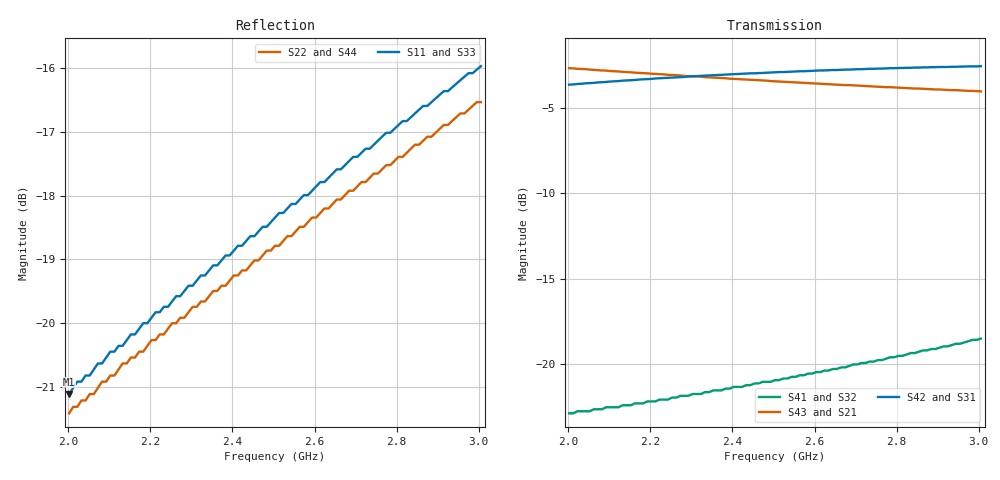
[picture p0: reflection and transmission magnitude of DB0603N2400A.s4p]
!	AVX THIN FILM OPERATION
!	0603 SIZE 3dB 90deg COUPLER P/N DB0603N2400ANTR
!	Created August 2007
!	Network Analyzer HP8720E S.07.64: Feb23, 2000 Serial No.US39172382
#	MHZ	S	MA	R	50
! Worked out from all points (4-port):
!   101 points, 2.003 GHz to 3.005 GHz, reference 50 ohm
!   strongest paths, dB at 2.003 GHz, 2.253 GHz, 2.504 GHz, 2.754 GHz, 3.005 GHz:
!     S42: -3.6, -3.2, -2.9, -2.7, -2.6
!     S31: -3.8, -3.4, -3.1, -3.0, -2.9
!     S43: -2.7, -3.1, -3.5, -3.8, -4.0
!     S21: -2.7, -3.1, -3.5, -3.8, -4.0
!     S41: -22.9, -21.9, -20.9, -19.7, -18.5
!     S32: -22.9, -21.9, -20.9, -19.7, -18.5
!   lowest |S11| = -21.1 dB at 2.003 GHz (marker M1), VSWR 1.19, Z = 48.2 + j8.47 ohm
!   |S11| at or under -10 dB: start of sweep to end of sweep
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2002.506  0.088 97.3  0.734 -49.8  0.647 39.6  0.072 57.6
          0.734 -49.8  0.085 103.6  0.072 57.6  0.657 39.4
          0.647 39.6  0.072 57.6  0.088 97.3  0.734 -49.8
          0.072 57.6  0.657 39.4  0.734 -49.8  0.085 103.6
2102.757  0.095 94.9  0.72 -51.5  0.66 38.0  0.075 58.3
          0.72 -51.5  0.091 101.6  0.075 58.3  0.671 37.8
          0.66 38.0  0.075 58.3  0.095 94.9  0.72 -51.5
          0.075 58.3  0.671 37.8  0.72 -51.5  0.091 101.6
2243.108  0.103 91.7  0.702 -53.8  0.675 35.8  0.079 59.3
          0.702 -53.8  0.099 98.9  0.079 59.3  0.688 35.6
          0.675 35.8  0.079 59.3  0.103 91.7  0.702 -53.8
          0.079 59.3  0.688 35.6  0.702 -53.8  0.099 98.9
2273.183  0.105 91.0  0.699 -54.2  0.678 35.4  0.081 59.5
          0.699 -54.2  0.101 98.4  0.081 59.5  0.691 35.1
          0.678 35.4  0.081 59.5  0.105 91.0  0.699 -54.2
          0.081 59.5  0.691 35.1  0.699 -54.2  0.101 98.4
2503.759  0.121 85.9  0.672 -57.8  0.696 32.1  0.09 61.0
          0.672 -57.8  0.115 94.4  0.09 61.0  0.714 31.8
          0.696 32.1  0.09 61.0  0.121 85.9  0.672 -57.8
          0.09 61.0  0.714 31.8  0.672 -57.8  0.115 94.4
2734.336  0.137 81.1  0.65 -61.3  0.708 29.1  0.102 61.9
          0.65 -61.3  0.13 90.7  0.102 61.9  0.731 28.6
          0.708 29.1  0.102 61.9  0.137 81.1  0.65 -61.3
          0.102 61.9  0.731 28.6  0.65 -61.3  0.13 90.7
3005.013  0.159 75.5  0.628 -65.3  0.714 25.9  0.119 62.0
          0.628 -65.3  0.149 86.5  0.119 62.0  0.744 25.2
          0.714 25.9  0.119 62.0  0.159 75.5  0.628 -65.3
          0.119 62.0  0.744 25.2  0.628 -65.3  0.149 86.5
